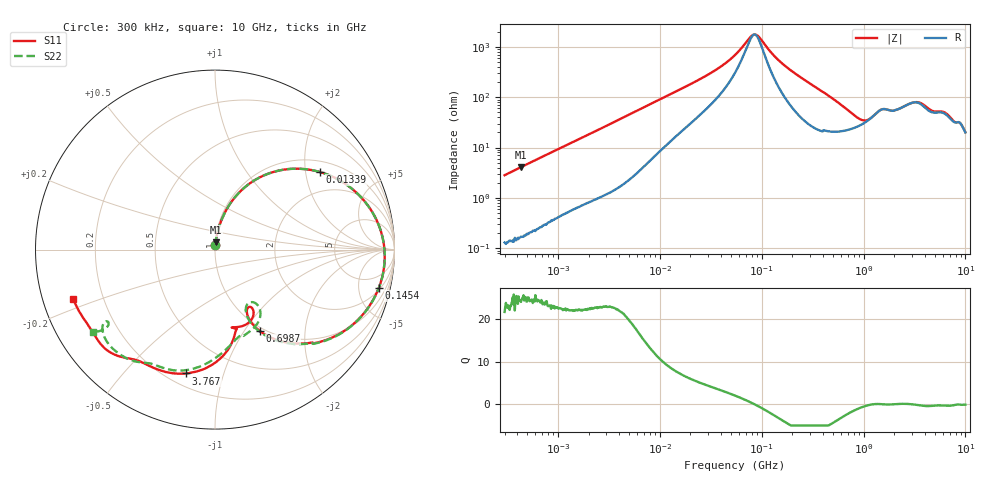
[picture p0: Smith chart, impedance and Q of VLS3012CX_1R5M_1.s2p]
! S-Parameter Data Generated by TDK Corporation
! Copyright(C) 2020 TDK Corporation.
! All Rights Reserved.
! TDK P/N: VLS3012CX-1R5M-1 (Inductor)
! Property: L=1.5uH at 1MHz
! Size(LxWxT): 3x3x1.2mm
! Model Type: s2p (Touchstone File Format Version 1.0)
! Frequency: DC=Yes Start=0.3MHz Stop=10000MHz 802points Log-sweep
! Model Generated on Aug. 18, 2020
! Port Assignments:
!  1 ---@@@--- 2
! Applicable Conditions:
!  Temperature = 25 degC
!  DC Bias Current = 0 A
!  Small Signal Operation
! Terms and conditions regarding TDK Simulation Models
! (1)This simulation model is being provided solely for informational purposes. Please refer to the specifications of the products in terms of detailed characteristics of such products.
! (2)In no event shall TDK Corporation of any of its subsidiaries be liable for any loss or damage arising, directly or indirectly,
!  From any information contained in this simulation model, including, but not limited to loss or damages arising from any inaccuracies, omissions or errors in connection with such information.
! (3)Any and all copyrights on this simulation model are owned by TDK Corporation.
!  Duplication or redistribution of this simulation model without prior written permission from TDK Corporation is prohibited.
! (4)This simulation model is subject to any modification or change without any prior notice.
! (5)Neither TDK Corporation nor any of its subsidiaries shall make any warranty, express or implied,
!  Including but not limited to the correctness, implied warranties of merchantability and fitness for a particular purpose with respect to this simulation models.
! (6)The use of this simulation model shall be deemed to have consented to the terms and conditions hereof.
# Hz S MA R 50
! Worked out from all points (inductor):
!   801 points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, 300 kHz to 10 GHz, reference 50 ohm
!   read as one part in series: L = 1.5 uH near 318.3 kHz
!   highest Q = 25 at 434.4 kHz (marker M1), where L = 1.5 uH
!   self-resonance near 84.86 MHz
!   S11 on the Smith chart (normalised r, x): 300 kHz: 1.00, +0.06; 13.39 MHz: 1.31, +2.41; 145.4 MHz: 2.28, -8.01; 698.7 MHz: 0.95, -1.18; 3.767 GHz: 0.27, -0.76; 10 GHz: 0.09, -0.17
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300000  0.02815 85.7  0.9984 -1.6  0.9982 -1.6  0.02795 85.8
434438  0.04054 85.1  0.9977 -2.3  0.9973 -2.3  0.04048 85.4
1713600  0.1528 78.6  0.9815 -8.8  0.9812 -8.8  0.1529 78.6
4363314  0.3593 66.1  0.9166 -21.2  0.9163 -21.2  0.3594 66.1
9671944  0.6292 45.7  0.7223 -39.1  0.7222 -39.1  0.6292 45.7
1.339226e7  0.7276 36.4  0.6035 -46.6  0.6034 -46.6  0.7277 36.4
3.118733e7  0.8867 16.1  0.2994 -60.4  0.2993 -60.4  0.8868 16.0
5.477226e7  0.9325 5.5  0.1356 -58.2  0.1356 -58.3  0.9326 5.4
7.683413e7  0.9447 -0.5  0.06143 -27.2  0.06143 -27.2  0.9448 -0.6
8.622688e7  0.9466 -2.6  0.05358 2.2  0.05358 2.2  0.9466 -2.7
1.454054e8  0.9371 -13.2  0.1684 59.5  0.1684 59.5  0.9372 -13.4
3.126428e8  0.8309 -35.0  0.4508 46.7  0.4507 46.7  0.8307 -35.3
4.687561e8  0.693 -49.0  0.6029 30.2  0.6028 30.2  0.6918 -49.5
6.987102e8  0.5183 -61.1  0.7066 10.4  0.7066 10.4  0.5144 -61.7
9.330971e8  0.4057 -63.6  0.7248 -5.5  0.7247 -5.5  0.3953 -63.9
1.228555e9  0.3771 -58.1  0.6709 -21.1  0.6709 -21.1  0.3563 -55.2
1.767019e9  0.451 -72.3  0.5696 -31.3  0.5698 -31.2  0.49 -64.8
2.798208e9  0.5641 -82.7  0.4455 -52.5  0.4456 -52.6  0.579 -86.3
3.766866e9  0.7087 -103.2  0.3569 -55.2  0.3567 -55.2  0.6932 -104.1
6.818311e9  0.8184 -135.8  0.2714 -78.1  0.2711 -78.0  0.7897 -133.4
8.211115e9  0.8222 -145.7  0.2374 -86.2  0.2371 -86.2  0.7335 -146.7
1e10  0.8357 -160.8  0.2249 -87.5  0.2244 -87.4  0.817 -146.0
